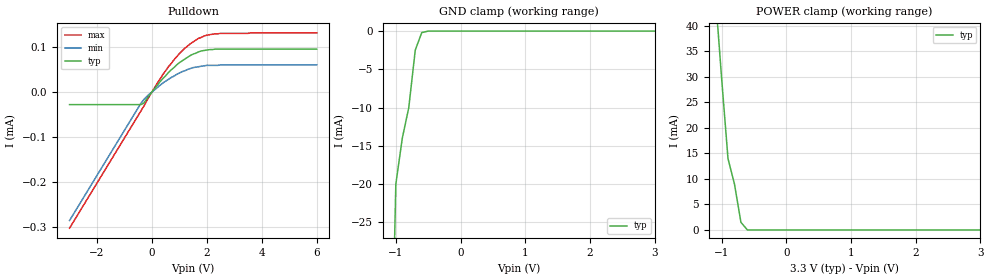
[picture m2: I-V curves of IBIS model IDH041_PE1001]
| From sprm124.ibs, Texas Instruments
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[Model]   IDH041_PE1001
Model_type   Input
Polarity   Non-Inverting
| signals
Vinl = 0.8V
Vinh = 2.0V
|   typ   min   max
C_comp   3.5490p   3.5093p   3.8191p
|   typ   min   max
[Temperature Range]   25.0   0   90
|   typ   min   max
[Voltage Range]   3.3V   3.13V   3.47V
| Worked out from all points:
|   slope of the pulldown table from 0 to 0.495 V, typ, clamps not added: 13.9 kohm
|   GND clamp passes 1 mA (typ) near -0.63 V on its own axis
|   POWER clamp passes 1 mA (typ) near -0.67 V on its own axis
[Pulldown]
|   Voltage   I(typ)   I(min)   I(max)
-3V       -28uA      -285uA     -302uA
-400mV    -28uA      -25uA      -42uA
-300mV    -25uA      -17uA      -32uA
200mV     15uA       10uA       20uA
600mV     43uA       28uA       56uA
1V        65uA       42uA       85uA
1.4V      81uA       52uA       107uA
1.7V      89uA       56uA       119uA
1.9V      92uA       58uA       124uA
2.3V      95uA       59uA       129uA
6V        95uA       60uA       131uA
[GND_clamp]
|   Voltage   I(typ)   I(min)   I(max)
-3V       -900mA     NA         NA
-2V       -400mA     NA         NA
-1V       -20mA      NA         NA
-900mV    -14mA      NA         NA
-800mV    -10mA      NA         NA
-700mV    -2.5mA     NA         NA
-600mV    -200uA     NA         NA
-500mV    0A         NA         NA
3V        0A         NA         NA
[POWER_clamp]
|   Voltage   I(typ)   I(min)   I(max)
-3V       600mA      NA         NA
-2V       200mA      NA         NA
-1V       30mA       NA         NA
-900mV    14mA       NA         NA
-800mV    9mA        NA         NA
-700mV    1.5mA      NA         NA
-600mV    0A         NA         NA
-500mV    0A         NA         NA
3V        0A         NA         NA
